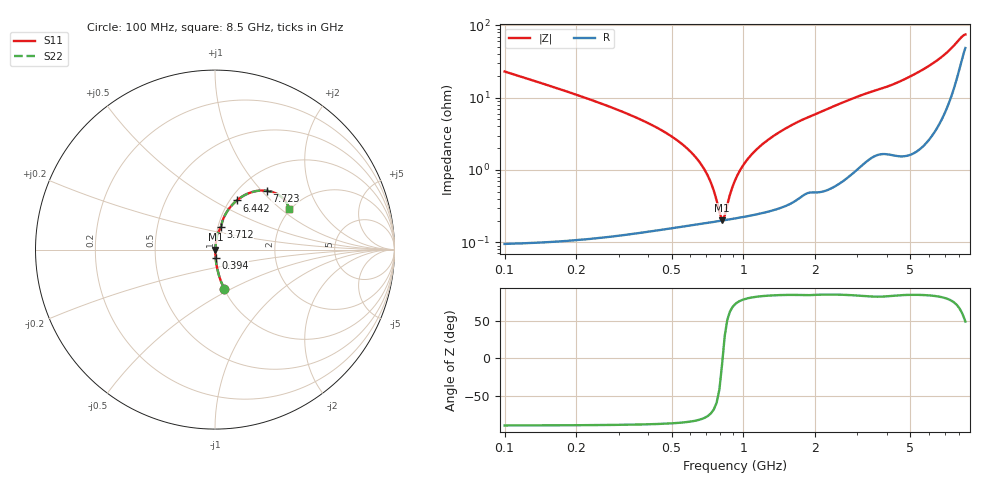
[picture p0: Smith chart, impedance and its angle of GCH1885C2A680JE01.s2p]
!Murata Part Number: GCH1885C2A680JE01
!These Parameters are Measured in Series Mode Connection
!Data Generated on Jun 19, 2026
!  o--ll--o
!Port1  Port2
!  o------o
!Operation Temp=25[degC], DC Bias Voltage=0[V]
!Freq. Start=100[MHz] Stop=9[GHz] 401[Steps]
# Hz S RI R 50
!Freq.(Hz) S11(Real) S11(Imag) S21(Real) S21(Imag) S12(Real) S12(Imag) S22(Real) S22(Imag)
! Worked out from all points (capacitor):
!   401 points, 100 MHz to 8.5 GHz, reference 50 ohm
!   read as one part in series: C = 68.1 pF near 142 MHz
!   lowest |Z| = 201 mohm at 814 MHz (marker M1)
!   series resonance near 818 MHz, so ESL is about 560 pH
!   S11 on the Smith chart (normalised r, x): 100 MHz: 1.00, -0.46; 394 MHz: 1.00, -0.09; 3.712 GHz: 1.03, +0.26; 6.442 GHz: 1.07, +0.65; 7.723 GHz: 1.32, +1.07; 8.5 GHz: 1.98, +1.14
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1e8  0.0512 -0.2184  0.9488 0.2184  0.9488 0.2184  0.0512 -0.2184
2.26e8  0.0101 -0.0944  0.9899 0.0944  0.9899 0.0944  0.0101 -0.0944
3.94e8  0.00344 -0.0452  0.9966 0.0452  0.9966 0.0452  0.00344 -0.0452
6.46e8  0.00195 -0.0135  0.998 0.0135  0.998 0.0135  0.00195 -0.0135
7.09e8  0.00192 -0.00813  0.9981 0.00813  0.9981 0.00813  0.00192 -0.00813
7.93e8  0.00197 -0.00175  0.998 0.00175  0.998 0.00175  0.00197 -0.00175
8.14e8  0.00199 -0.000272  0.998 0.000272  0.998 0.000272  0.00199 -0.000272
8.56e8  0.00205 0.00258  0.9979 -0.00258  0.9979 -0.00258  0.00205 0.00258
9.19e8  0.00217 0.00663  0.9978 -0.00663  0.9978 -0.00663  0.00217 0.00663
9.61e8  0.00227 0.0092  0.9977 -0.0092  0.9977 -0.0092  0.00227 0.0092
1.066e9  0.00256 0.0152  0.9974 -0.0152  0.9974 -0.0152  0.00256 0.0152
1.255e9  0.00326 0.0252  0.9967 -0.0252  0.9967 -0.0252  0.00326 0.0252
1.507e9  0.00458 0.0374  0.9954 -0.0374  0.9954 -0.0374  0.00458 0.0374
2.116e9  0.00895 0.063  0.991 -0.063  0.991 -0.063  0.00895 0.063
2.914e9  0.0187 0.0964  0.9813 -0.0964  0.9813 -0.0964  0.0187 0.0964
3.712e9  0.032 0.1241  0.968 -0.1241  0.968 -0.1241  0.032 0.1241
4.3e9  0.0381 0.1473  0.9619 -0.1473  0.9619 -0.1473  0.0381 0.1473
5.707e9  0.0766 0.2257  0.9234 -0.2257  0.9234 -0.2257  0.0766 0.2257
6.442e9  0.121 0.2736  0.879 -0.2736  0.879 -0.2736  0.121 0.2736
7.114e9  0.1895 0.3148  0.8105 -0.3148  0.8105 -0.3148  0.1895 0.3148
7.723e9  0.2871 0.3281  0.7129 -0.3281  0.7129 -0.3281  0.2871 0.3281
8.5e9  0.4137 0.2244  0.5863 -0.2244  0.5863 -0.2244  0.4137 0.2244
